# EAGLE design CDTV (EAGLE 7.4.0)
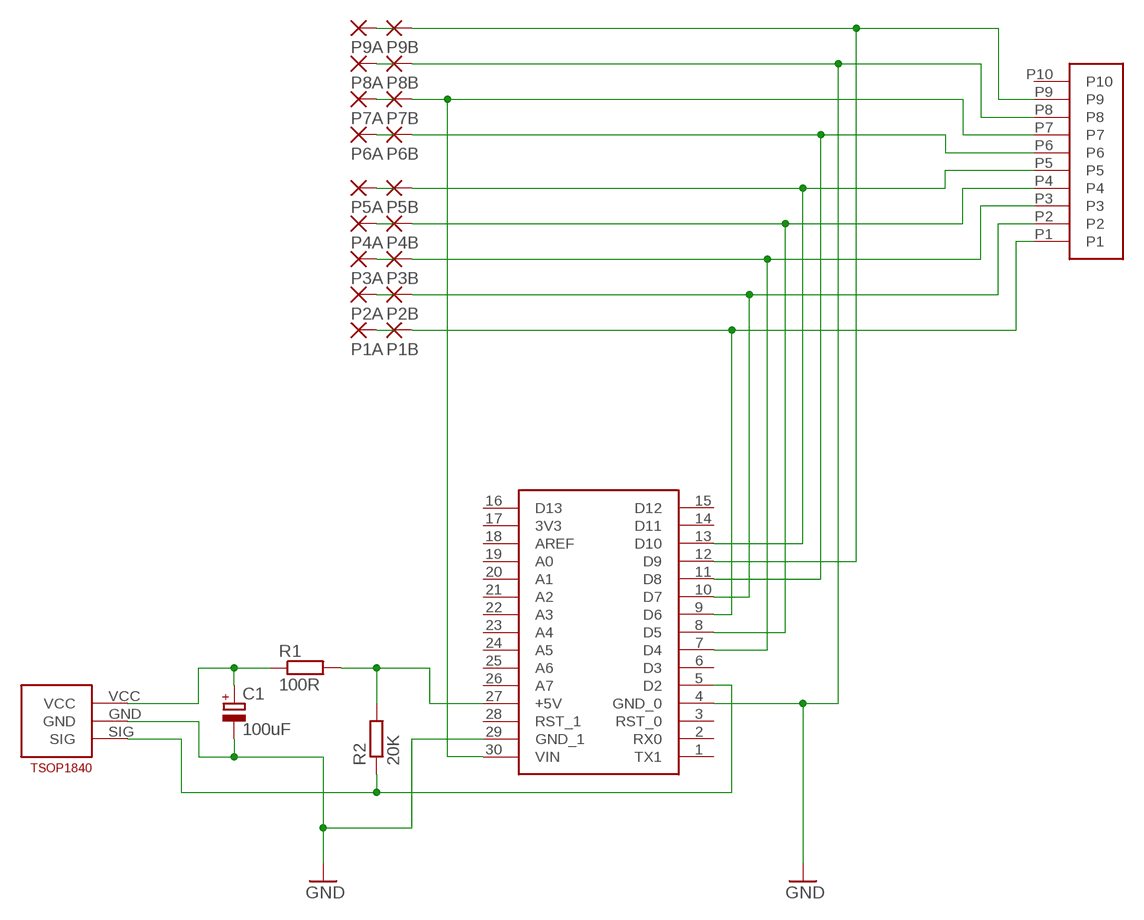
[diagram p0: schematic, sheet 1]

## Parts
ATMEGA328P  ARDUINO_NANO_V3  [ARDUINO_NANO_V3]
C1  100uF  CPOL-EUE2.5-5  [E2,5-5]
P1A  SMD2  [SMD1,27-2,54]
P1B  SMD2  [SMD1,27-2,54]
P2A  SMD2  [SMD1,27-2,54]
P2B  SMD2  [SMD1,27-2,54]
P3A  SMD2  [SMD1,27-2,54]
P3B  SMD2  [SMD1,27-2,54]
P4A  SMD2  [SMD1,27-2,54]
P4B  SMD2  [SMD1,27-2,54]
P5A  SMD2  [SMD1,27-2,54]
P5B  SMD2  [SMD1,27-2,54]
P6A  SMD2  [SMD1,27-2,54]
P6B  SMD2  [SMD1,27-2,54]
P7A  SMD2  [SMD1,27-2,54]
P7B  SMD2  [SMD1,27-2,54]
P8A  SMD2  [SMD1,27-2,54]
P8B  SMD2  [SMD1,27-2,54]
P9A  SMD2  [SMD1,27-2,54]
P9B  SMD2  [SMD1,27-2,54]
R1  100R  R-EU_0204/7  [0204/7]
R2  20K  R-EU_0204/7  [0204/7]
TSOP1840  TSOP1838  [TSOP1838]
U$1  JOYJACK  [JOYJACK]

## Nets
GND: ATMEGA328P.4(GND_0) ATMEGA328P.29(GND_1) C1.- P8B.1(P) TSOP1840.GND U$1.P8
N$1 [vcc]: ATMEGA328P.27(+5V) R1.2 R2.2
N$2 [vcc]: C1.+ R1.1 TSOP1840.VCC
N$3: P6A.1(P)
N$4: ATMEGA328P.9(D6) P1B.1(P) U$1.P1
N$5: ATMEGA328P.10(D7) P2B.1(P) U$1.P2
N$6: ATMEGA328P.7(D4) P3B.1(P) U$1.P3
N$7: ATMEGA328P.8(D5) P4B.1(P) U$1.P4
N$8: ATMEGA328P.13(D10) P5B.1(P) U$1.P5
N$9: ATMEGA328P.11(D8) P6B.1(P) U$1.P6
N$10 [power]: ATMEGA328P.30(VIN) P7B.1(P) U$1.P7
N$11: P1A.1(P)
N$12: P2A.1(P)
N$13: P3A.1(P)
N$14: P4A.1(P)
N$15: P5A.1(P)
N$16: P7A.1(P)
N$17: P8A.1(P)
N$18: P9A.1(P)
N$20: ATMEGA328P.12(D9) P9B.1(P) U$1.P9
SIG [vcc]: ATMEGA328P.5(D2) R2.1 TSOP1840.SIG
Unconnected: ATMEGA328P.1(TX1) ATMEGA328P.2(RX0) ATMEGA328P.3(RST_0) ATMEGA328P.6(D3) ATMEGA328P.14(D11) ATMEGA328P.15(D12) ATMEGA328P.16(D13) ATMEGA328P.17(3V3) ATMEGA328P.18(AREF) ATMEGA328P.19(A0) ATMEGA328P.20(A1) ATMEGA328P.21(A2) ATMEGA328P.22(A3) ATMEGA328P.23(A4) ATMEGA328P.24(A5) ATMEGA328P.25(A6) ATMEGA328P.26(A7) ATMEGA328P.28(RST_1) U$1.P10

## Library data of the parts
ATMEGA328P = arduino_nano_v3:ARDUINO_NANO_V3: Arduino Nano v3
C1 = rcl:CPOL-EU: POLARIZED CAPACITOR, European symbol
P1A P1B P2A P2B P3A P3B P4A P4B P5A P5B P6A P6B P7A P7B P8A P8B P9A P9B = wirepad:SMD2: SMD PAD
R1 R2 = rcl:R-EU_: RESISTOR, European symbol
TSOP1840 = TSOP1840:TSOP1838: IR Receiver (TSOP1840)
U$1 = joy_jack:JOYJACK: Joystick (Pin Header)

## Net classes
0 default: width 0.406 mm, clearance 0.152 mm
1 vcc: width 0.61 mm, clearance 0.203 mm
2 power: width 0.813 mm, clearance 0.254 mm

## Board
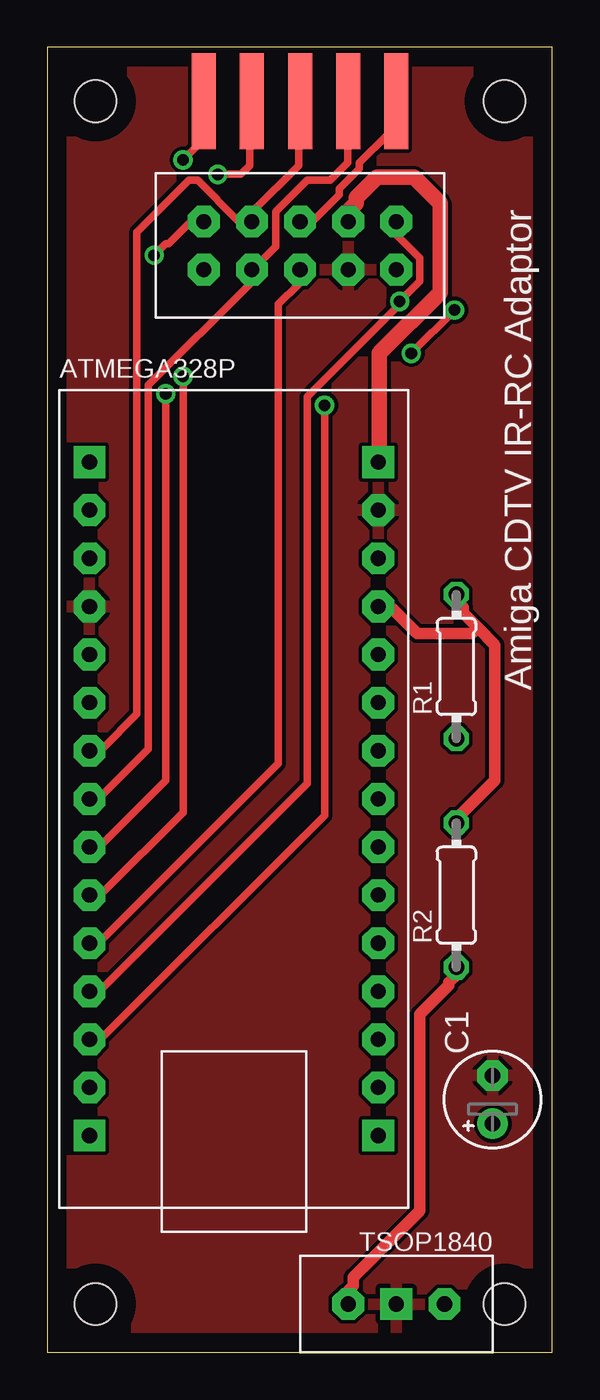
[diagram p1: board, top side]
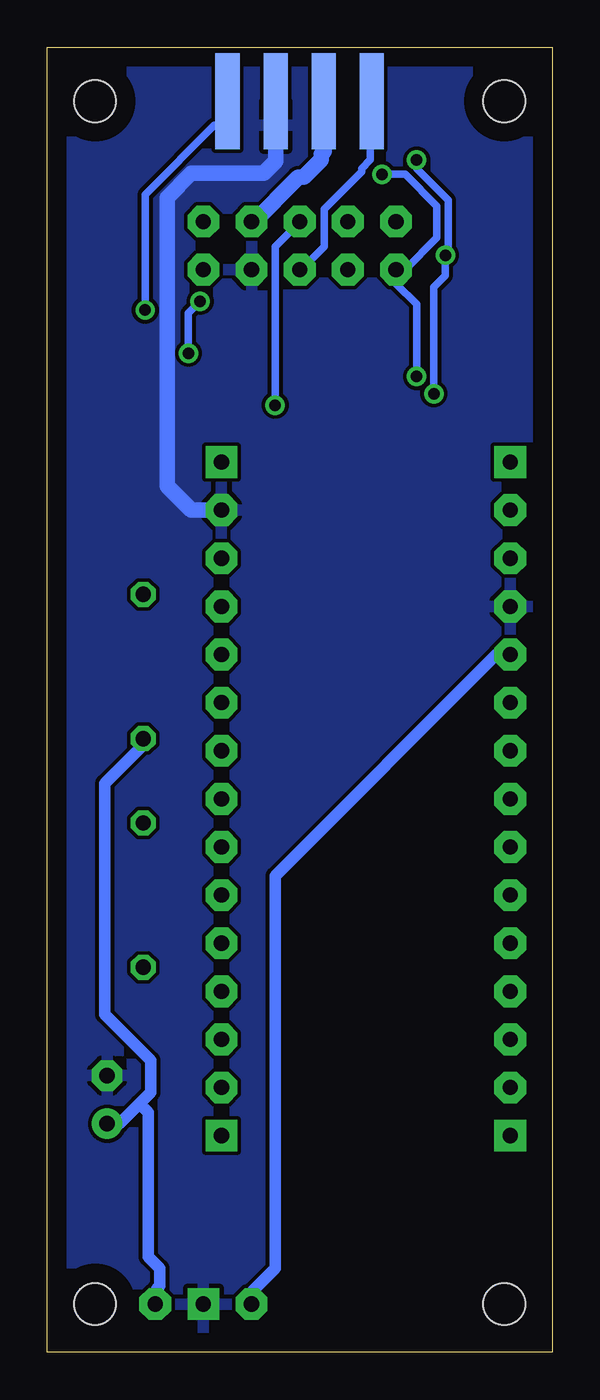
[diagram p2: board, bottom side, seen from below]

Size 26.65 x 68.89 mm. Coordinates in mm from the lower left corner, seen from the top.
Outline: 0,0 26.65,0 26.65,68.89 0,68.89 0,0
Copper layers (1*16): Top 0.035mm / dielectric 1.5mm / Bottom 0.035mm
Design rules "default": minimum track width 10mil, minimum drill 24mil, track to track 8mil, track to pad 8mil, pad to pad 8mil, via to via 8mil, smd to smd 8mil, copper to edge 40mil, drill to drill 8mil, minimum pad ring 10mil, minimum via ring 8mil, stop-mask expansion 4mil, vias tented up to drill 0mil, thermal gap 10mil
Holes 2.2 mm at 2.54,2.54 2.54,66.04 24.13,66.04 24.13,2.54

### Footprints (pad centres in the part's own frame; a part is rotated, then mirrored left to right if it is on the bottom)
ARDUINO_NANO_V3 = drill 0.8 pad 1.676 square: 1 17.78,7.938; 15 -17.78,7.938; 16 -17.78,-7.303; 30 17.78,-7.303 | drill 0.8 pad 1.676 octagon: 2 15.24,7.938; 3 12.7,7.938; 4 10.16,7.938; 5 7.62,7.938; 6 5.08,7.938; 7 2.54,7.938; 8 0,7.938; 9 -2.54,7.938; 10 -5.08,7.938; 11 -7.62,7.938; 12 -10.16,7.938; 13 -12.7,7.938; 14 -15.24,7.938; 17 -15.24,-7.303; 18 -12.7,-7.303; 19 -10.16,-7.303; 20 -7.62,-7.303; 21 -5.08,-7.303; 22 -2.54,-7.303; 23 0,-7.303; 24 2.54,-7.303; 25 5.08,-7.303; 26 7.62,-7.303; 27 10.16,-7.303; 28 12.7,-7.303; 29 15.24,-7.303
E2,5-5 = drill 0.813 pad 1.6: + -1.27,0 | drill 0.813 pad 1.6 octagon: - 1.27,0
SMD1,27-2,54 = smd 1.27 x 2.54: 1 0,0
0204/7 = drill 0.813 octagon: 1 -3.81,0; 2 3.81,0
TSOP1838 = drill 0.8 pad 1.676 square: GND 0,0 | drill 0.8 pad 1.676 octagon: SIG -2.54,0; VCC 2.54,0
JOYJACK = drill 0.8 pad 1.676 octagon: P1 0,2.54; P2 0,0; P3 2.54,2.54; P4 2.54,0; P5 5.08,2.54; P6 5.08,0; P7 7.62,2.54; P8 7.62,0; P9 10.16,2.54; P10 10.16,0

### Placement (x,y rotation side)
ATMEGA328P  10.16,29.21 90 top
C1  23.5,13.34 90 top
P1A  8.26,67.31 180 top
P1B  8.26,64.77 180 top
P2A  10.79,67.31 180 top
P2B  10.79,64.77 180 top
P3A  13.34,67.31 180 top
P3B  13.34,64.77 180 top
P4A  15.88,67.31 180 top
P4B  15.88,64.77 180 top
P5A  18.41,67.31 180 top
P5B  18.41,64.77 180 top
P6A  9.53,67.31 0 bottom
P6B  9.53,64.77 0 bottom
P7A  12.06,67.31 0 bottom
P7B  12.06,64.77 0 bottom
P8A  14.61,67.31 0 bottom
P8B  14.61,64.77 0 bottom
P9A  17.14,67.31 0 bottom
P9B  17.14,64.77 0 bottom
R1  21.59,36.2 90 top
R2  21.59,24.13 90 top
TSOP1840  18.41,2.54 0 top
U$1  8.26,57.15 0 top

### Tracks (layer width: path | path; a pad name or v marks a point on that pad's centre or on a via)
GND
  Bottom 0.813: ATMEGA328P.29 19.05,44.45 20.32,45.72 20.32,60.96 19.05,62.23 15.24,62.23 14.61,62.87 P8B.1
  pour Top: 0,68.58 0,0 26.67,0 26.67,68.58
  pour Bottom: 0,68.58 0,0 26.67,0 26.67,68.58
N$1
  Top 0.61: 22.71,38.25 21.95,39.01 21.95,39.32 21.64,39.62 21.64,39.93 R1.2 | 22.71,38.25 23.62,37.34 23.62,30.18 21.64,28.19 21.64,28.04 R2.2 | ATMEGA328P.27 17.53,39.32 18.14,39.32 19.51,37.95 22.4,37.95 22.71,38.25
N$2
  Bottom 0.61: 21.79,13.11 22.86,12.04 23.47,12.04 C1.+ | 21.79,13.11 21.18,13.72 21.18,15.39 23.62,17.83 23.62,30.02 21.64,32 21.64,32.31 R1.1 | 21.79,13.11 21.34,12.65 21.34,5.03 20.73,4.42 20.73,3.5 20.88,3.35 20.88,2.59 TSOP1840.VCC
N$4  (via drill 0.61)
  Top 0.406: v7.16,62.94 8.23,64.01 8.23,64.77 P1B.1 | v5.64,57.91 6.25,58.52 6.4,58.52 7.47,59.59 8.23,59.59 U$1.P1 | ATMEGA328P.9 2.74,26.67 6.25,30.18 v6.25,50.6
  Bottom 0.406: v7.16,62.94 7.16,62.48 5.49,60.81 5.49,58.06 v5.64,57.91 5.64,56.84 6.25,56.24 v6.25,50.6
N$5  (via drill 0.61)
  Top 0.406: v8.99,62.18 10.21,62.18 10.67,62.64 10.67,64.77 P2B.1 | v7.16,51.51 7.16,28.5 2.9,24.23 2.29,24.23 ATMEGA328P.10
  Bottom 0.406: v8.99,62.18 7.77,62.18 6.1,60.5 6.1,58.83 7.77,57.15 U$1.P2 8.23,57 8.23,56.39 7.16,55.32 v7.16,51.51
N$6
  Top 0.406: P3B.1 13.26,64.77 13.26,62.64 10.82,60.2 10.82,59.74 U$1.P3 10.67,59.74 10.06,59.74 7.92,61.87 7.47,61.87 4.72,59.13 4.72,33.68 2.9,31.85 2.29,31.85 ATMEGA328P.7
N$7
  Top 0.406: P4B.1 15.85,64.77 15.85,62.79 14.94,61.87 13.72,61.87 12.04,60.2 12.04,58.37 10.82,57.15 U$1.P4 10.67,57 10.67,56.39 5.33,51.05 5.33,31.85 2.74,29.26 2.29,29.26 ATMEGA328P.8
N$8  (via drill 0.61)
  Top 0.406: P5B.1 18.29,64.77 17.98,64.47 17.98,64.31 16.46,62.79 16.46,62.48 15.39,61.42 15.39,61.11 14.02,59.74 13.41,59.74 U$1.P5 | v14.63,49.99 14.63,28.35 2.9,16.61 2.29,16.61 ATMEGA328P.13
  Bottom 0.406: v14.63,49.99 14.63,58.37 13.41,59.59 U$1.P5
N$9
  Top 0.406: ATMEGA328P.11 2.29,21.64 2.74,21.64 12.19,31.09 12.19,55.32 13.26,56.39 13.26,57.15 U$1.P6
  Bottom 0.406: P6B.1 9.6,64.77 9.6,62.94 10.06,62.48 10.06,62.33 12.04,60.35 12.04,58.37 13.26,57.15 U$1.P6
N$10
  Top 0.813: ATMEGA328P.30 17.53,47.09 17.53,52.73 20.73,55.93 20.73,60.66 19.36,62.03 17.37,62.03 16.31,60.96 16.31,60.66 15.85,60.2 15.85,59.74 U$1.P7
  Bottom 0.813: P7B.1 12.04,64.77 12.04,63.4 12.19,63.25 12.19,62.94 13.11,62.03 13.41,62.03 15.85,59.59 U$1.P7
N$20  (via drill 0.61)
  Top 0.406: v19.2,52.73 v21.49,55.02 | U$1.P9 18.44,59.59 18.44,58.98 19.66,57.76 19.66,56.54 v18.59,55.47 18.59,55.32 13.72,50.44 13.72,30.02 2.74,19.05 ATMEGA328P.12
  Bottom 0.406: P9B.1 17.83,64.77 21.49,61.11 v21.49,55.02 | v19.2,52.73 19.2,54.86 v18.59,55.47
SIG
  Top 0.61: R2.1 21.49,20.27 21.49,19.81 21.18,19.51 21.18,19.36 19.66,17.83 19.66,7.47 16.15,3.96 16.15,3.5 15.85,3.2 15.85,2.59 TSOP1840.SIG
  Bottom 0.61: ATMEGA328P.5 2.29,36.88 2.9,36.88 14.63,25.15 14.63,4.42 15.85,3.2 15.85,2.59 TSOP1840.SIG

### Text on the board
tPlace: ATMEGA328P
tNames: Amiga CDTV IR-RC Adaptor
